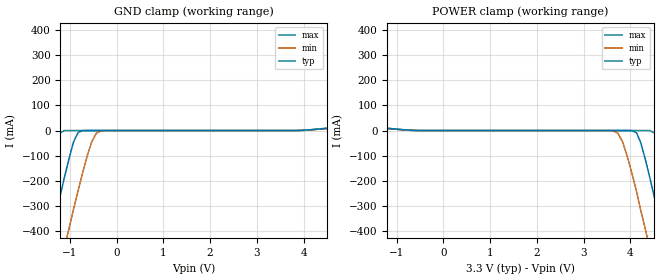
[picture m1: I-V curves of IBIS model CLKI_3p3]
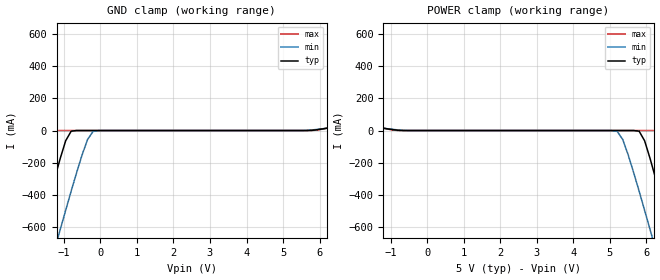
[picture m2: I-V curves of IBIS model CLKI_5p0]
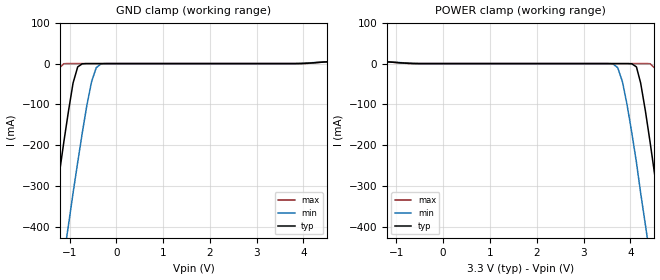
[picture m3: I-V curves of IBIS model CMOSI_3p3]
|   Texas Instruments Incorporated
|   IBIS Model of ADC128S102-SEP
[IBIS Ver]   4.2
[File name]   adc128s102-sep.ibs
[File Rev]   1.1   | Initial Release
[Notes]
Created By  Pegah Alavi
   Rev1.0 : Initial Release
   Rev1.1 : Added models for Vdd = 5V
This model supports the LVCMOS Input, LVCMOS Output, Clock input, and SPI
pins. All of these pins are modeled with supply voltage of 3.3V and 5.0V.
The default supply voltage is 3.3V. Model Selector is used to switch
between the two supply conditions. Analog and other pins are not modeled.
Begin IBIS Parser Results
| Do NOT edit this section manually!
...\ADC128s102-sep.ibs for IBIS 4.2 Compatibility...
Errors  : 0
File Passed
| End IBIS Parser Results
[Date]   03/28/2022
[Source]
[Disclaimer]
| This model is designed as an aid for customers of Texas Instruments.
| TI and its licensors and suppliers make no warranties, either expressed
| or implied, with respect to this model, including the warranties of
| merchantability or fitness for a particular purpose. The model is
| provided solely on an "as is" basis. The entire risk as to its quality
| and performance is with the customer.
| This model is subject to change without notice. Texas Instruments
| Incorporated is not responsible for updating this model.
[Copyright]  Copyright 2022, Texas Instruments, All Rights Reserved
[Component]  ADC128S102-SEP
[Manufacturer]  Texas Instruments Corp
[Package]
|   typ   min   max
R_pkg   0   NA   NA
L_pkg   0   NA   NA
C_pkg   0   NA   NA
[Pin]   signal_name   model_name   R_pin   L_pin   C_pin
1   CS_B   SPI_X
2   VA   POWER
3   AGND   GND
4   IN0   NC
5   IN1   NC
6   IN2   NC
7   IN3   NC
8   IN4   NC
9   IN5   NC
10   IN6   NC
11   IN7   NC
12   DGND   GND
13   VD   POWER
14   DIN   CMOSI_X
15   DOUT   CMOSO_X
16   SCLK   CLKI_X
[Package Model] TSSOP16_PW
[Model Selector]   CLKI_X
CLKI_3p3   Clock Input with VDD=3.3V
CLKI_5p0   Clock Input with VDD=5.0V
[Model Selector]   CMOSI_X
CMOSI_3p3   CMOS Input with VDD=3.3V
CMOSI_5p0   CMOS Input with VDD=5.0V
[Model Selector]   CMOSO_X
CMOSO_3p3   CMOS Output with VDD=3.3V
CMOSO_5p0   CMOS Output with VDD=5.0V
[Model Selector]   SPI_X
SPI_3p3   SPI Input with VDD=3.3V
SPI_5p0   SPI Input with VDD=5.0V
[Define Package Model]  TSSOP16_PW
[Manufacturer] Texas Instruments
[OEM] NA
[Description]  Package model at 500MHz
[Number Of Pins]  16
[Pin Numbers]
1   | 1 = L1
2   | 2 = L2
3   | 3 = L3
4   | 4 = L4
5   | 5 = L5
6   | 6 = L6
7   | 7 = L7
8   | 8 = L8
9   | 9 = L9
10   | 10 = L10
11   | 11 = L11
12   | 12 = L12
13   | 13 = L13
14   | 14 = L14
15   | 15 = L15
16   | 16 = L16
[Model Data]
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[End Model Data]
[End Package Model]
| Models and submodels in the file (8): CLKI_3p3 (Input), CLKI_5p0 (Input), CMOSI_3p3 (Input), CMOSI_5p0 (Input), SPI_3p3 (Input), SPI_5p0 (Input), CMOSO_3p3 (Output), CMOSO_5p0 (Output)
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|   Model CLKI_3p3
[Model]  CLKI_3p3
Model_type Input
Polarity   Non-Inverting
Vinl = 0
Vinh = 3.3
C_comp   102fF   98fF   106fF
[Temperature Range]   25.000   105.0   -40.0
[Voltage Range]   3.3   3.000   3.60
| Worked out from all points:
|   GND clamp passes 1 mA (typ) near -0.73 V on its own axis
|   POWER clamp passes 1 mA (typ) near -0.67 V on its own axis
[Power Clamp]
|Voltage   I(typ)   I(min)   I(max)
-3.3V     620mA      593mA      666mA
-2.71V    391mA      399mA      390mA
-1.82V    61.4mA     117mA      22.8mA
-1.32V    10.5mA     9.61mA     11.8mA
3.63V     -280pA     -1.06mA    -7.03pA
3.83V     -344nA     -44mA      -7.93pA
4.13V     -8.16mA    -242mA     -281pA
4.32V     -115mA     -394mA     -2.67uA
4.42V     -191mA     -472mA     -257uA
4.72V     -440mA     -710mA     -144mA
5.02V     -698mA     -952mA     -411mA
6.6V      -2.11A     -2.26A     -1.92A
[Gnd Clamp]
|Voltage   I(typ)   I(min)   I(max)
-3.3V     -2.11A     -2.26A     -1.92A
-1.72V    -698mA     -952mA     -411mA
-1.42V    -440mA     -710mA     -144mA
-1.12V    -191mA     -472mA     -257uA
-1.02V    -115mA     -394mA     -2.67uA
-825mV    -8.16mA    -242mA     -281pA
-528mV    -344nA     -44mA      -7.93pA
-330mV    -280pA     -1.06mA    -7.03pA
4.62V     10.5mA     9.61mA     11.8mA
5.12V     61.4mA     117mA      22.8mA
6.01V     391mA      399mA      390mA
6.6V      620mA      593mA      666mA
|   Model CLKI_5p0
[Model]  CLKI_5p0
Model_type Input
Polarity   Non-Inverting
Vinl = 0
Vinh = 5.0
C_comp   102fF   98fF   106fF
[Temperature Range]   25.000   105.0   -40.0
[Voltage Range]   5.0   4.50   5.50
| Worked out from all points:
|   GND clamp passes 1 mA (typ) near -0.68 V on its own axis
|   POWER clamp passes 1 mA (typ) near -0.75 V on its own axis
[Power Clamp]
|Voltage   I(typ)   I(min)   I(max)
-5V       1.95A      1.81A      2.11A
-2.9V     701mA      720mA      687mA
-2.75V    613mA      643mA      587mA
-2V       183mA      265mA      102mA
-1.55V    27.6mA     58mA       31mA
5.2V      -13.2pA    -5.65mA    -9.65pA
5.8V      -4.3mA     -376mA     -12.2pA
6.1V      -174mA     -615mA     -8.85nA
6.4V      -423mA     -857mA     -5.69mA
6.7V      -684mA     -1.1A      -215mA
7.15V     -1.08A     -1.47A     -630mA
10V       -3.64A     -3.85A     -3.37A
[Gnd Clamp]
|Voltage   I(typ)   I(min)   I(max)
-5V       -3.64A     -3.85A     -3.37A
-2.15V    -1.08A     -1.47A     -630mA
-1.7V     -684mA     -1.1A      -215mA
-1.4V     -423mA     -857mA     -5.69mA
-1.1V     -174mA     -615mA     -8.85nA
-800mV    -4.3mA     -376mA     -12.2pA
-200mV    -13.2pA    -5.65mA    -9.65pA
6.55V     27.6mA     58mA       31mA
7V        183mA      265mA      102mA
7.75V     613mA      643mA      587mA
7.9V      701mA      720mA      687mA
10V       1.95A      1.81A      2.11A
|   Model CMOSI_3p3
[Model]  CMOSI_3p3
Model_type Input
Polarity   Non-Inverting
Vinl = 0
Vinh = 3.3
C_comp   131.2fF   130.5fF   132fF
[Temperature Range]   25.000   105.00   -40.000
[Voltage Range]   3.300V   3.000V   3.600V
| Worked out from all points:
|   GND clamp passes 1 mA (typ) near -0.73 V on its own axis
|   POWER clamp passes 1 mA (typ) near -0.79 V on its own axis
[Power Clamp]
|Voltage   I(typ)   I(min)   I(max)
-3.3V     70.7mA     31mA       84mA
-1.72V    9.31mA     8.51mA     10.2mA
3.63V     -280pA     -1.06mA    -7.16pA
3.83V     -344nA     -44mA      -8.05pA
4.13V     -8.16mA    -242mA     -281pA
4.32V     -115mA     -394mA     -2.67uA
4.42V     -191mA     -472mA     -257uA
4.52V     -272mA     -551mA     -10.7mA
4.62V     -355mA     -631mA     -65.2mA
4.72V     -440mA     -710mA     -144mA
5.02V     -698mA     -952mA     -411mA
6.6V      -2.11A     -2.26A     -1.92A
[Gnd Clamp]
|Voltage   I(typ)   I(min)   I(max)
-3.3V     -2.11A     -2.26A     -1.92A
-1.72V    -698mA     -952mA     -411mA
-1.42V    -440mA     -710mA     -144mA
-1.22V    -272mA     -551mA     -10.7mA
-1.12V    -191mA     -472mA     -257uA
-1.02V    -115mA     -394mA     -2.67uA
-924mV    -47.6mA    -317mA     -26.9nA
-825mV    -8.16mA    -242mA     -281pA
-528mV    -344nA     -44mA      -8.05pA
-330mV    -280pA     -1.06mA    -7.16pA
5.02V     9.31mA     8.51mA     10.2mA
6.6V      70.7mA     31mA       84mA
